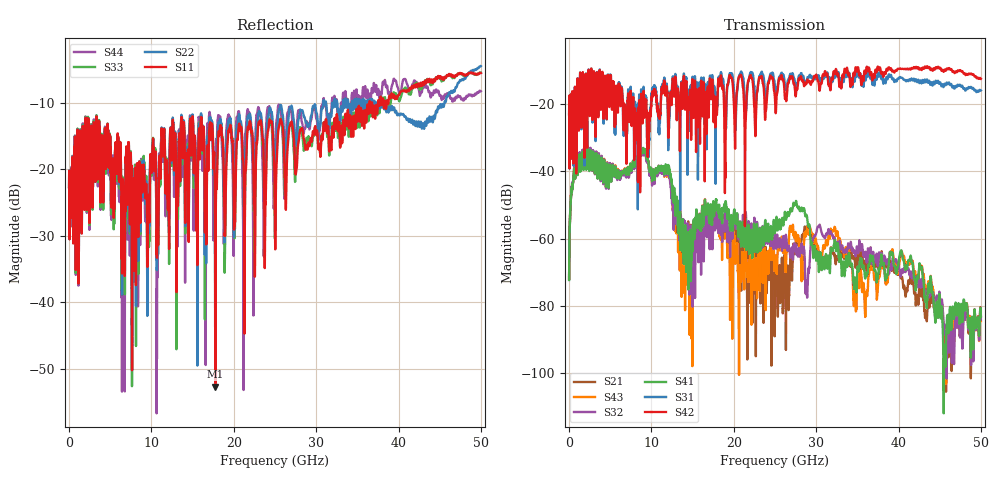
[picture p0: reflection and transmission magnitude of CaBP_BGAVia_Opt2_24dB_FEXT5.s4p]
!* Samtec Inc. NovaRay Examax Flyover System  *
!*  REV DATE  = 08/08/18  *
!*  TYPE  = TOUCHSTONE  *
!*  PORTS  = 4 port  *
!*  UNITS  = GHz  *
!*  DATA RANGE = DC  to 50 GHz; 10 MHz Step  *
!*  PARAMETER  = S  *
!*  FORMAT  = Real-Imaginary  *
!*  REFERENCE  = 50 ohms  *
!*  SOURCE  = HFSS  *
!*  VALIDATED  = No  *
!*  MANUFACTURER = SAMTEC  *
!*  INTERCONNECT = NVAx to EBCx to EBCx to NVAx  *
!*  [Full Channel NVAx to EBCx to EBCx to NVAx  with PCB Trace and BGA Via]  *
!*  BOUNDARY A  = Silicon BGA Ball Pad  *
!*  BOUNDARY B  = Silicon BGA Ball Pad  *
!*  NVAx (end a) ->>- (end b) NVAx  *
!*  Port 01 ->>- Port 02  *
!*  Port 03 ->>- Port 04  *
!***************************** CHANNEL MODEL ******************************************
# GHz S RI R 50
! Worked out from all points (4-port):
!   5000 points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, 10 MHz to 50 GHz, reference 50 ohm
!   strongest paths, dB at 10 MHz, 12.51 GHz, 25.01 GHz, 37.51 GHz, 50 GHz:
!     S42: -23.2, -15.0, -19.0, -9.0, -12.6
!     S31: -23.2, -14.5, -15.2, -10.7, -16.0
!     S41: -72.3, -45.9, -57.4, -71.1, -83.2
!     S32: -71.7, -49.7, -59.0, -67.6, -84.0
!     S43: -71.9, -48.6, -67.3, -73.4, -84.5
!     S21: -72.0, -47.5, -72.3, -68.1, -83.0
!   lowest |S11| = -52.7 dB at 17.77 GHz (marker M1), VSWR 1.00, Z = 49.8 - j0.145 ohm
!   |S11| at or under -10 dB: start of sweep to 36.46 GHz; 36.55 GHz to 36.75 GHz (204 MHz wide, 0.557 % of centre); 36.79 GHz to 37.51 GHz (722.9 MHz wide, 1.95 % of centre)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
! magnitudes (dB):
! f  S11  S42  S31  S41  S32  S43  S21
! 10 MHz  -22.7  -23.2  -23.2  -72.3  -71.7  -71.9  -72.0
! 1.74 GHz  -13.6  -11.6  -11.8  -38.4  -37.6  -37.9  -38.0
! 11.92 GHz  -24.3  -16.7  -16.2  -39.3  -40.0  -40.2  -39.5
! 14.76 GHz  -12.9  -16.1  -14.5  -59.7  -59.6  -66.1  -58.8
! 17.77 GHz  -52.7  -26.6  -28.1  -50.4  -56.3  -53.4  -53.7
! 20.73 GHz  -13.7  -11.8  -11.4  -55.1  -55.3  -67.8  -57.9
! 50 GHz  -5.5  -12.6  -16.0  -83.2  -84.0  -84.5  -83.0
